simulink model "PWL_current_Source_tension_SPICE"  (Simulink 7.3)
settings: Solver=ode15s  StartTime=0.0  StopTime=10  RelTol=1e-3
StopFcn:
  | load signaux.mat
  | plotyy(x(1,:),x(2,:),x(1,:),x(3,:))
  | title('Dérivateur commandé par PWL Current et source I-->V')
  | xlabel('temps')
  | grid
  | gtext('Tension d''entrée')
  | gtext('Sortie du dérivateur')
libraries: fl_lib x10, nesl_utility x3, elec_lib x2

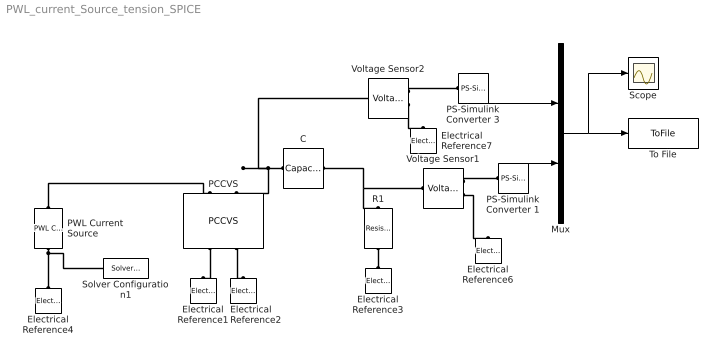
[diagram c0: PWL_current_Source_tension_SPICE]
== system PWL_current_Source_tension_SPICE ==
  C : fl_lib/Electrical/Electrical Elements/Capacitor  DialogController=NetworkEngine.DynNeDlgSource  SystemSampleTime=-1  c=1e-6 F  v0=0 V  r=0 Ohm  g=0 1/Ohm  i_Log=off  v_Log=off  vc_Log=off  LocalVarNames=|i|v|vc  LocalVarDescs=|i|v|Internal variable for voltage across capacitor term  LocalVarLogging=[0 0 0]
  Electrical Reference{1..4,6..7} (6 alike) : fl_lib/Electrical/Electrical Elements/Electrical Reference  DialogController=NetworkEngine.DynNeDlgSource  SystemSampleTime=-1  i_Log=off  LocalVarNames=|i  LocalVarDescs=|i  LocalVarLogging=[]
  Mux : Mux  Inputs=2
  PCCVS : elec_lib/Sources/SPICE-Compatible Sources/PCCVS  DialogController=NetworkEngine.DynNeDlgSource  SystemSampleTime=-1  PEES=[0 1 ]  LocalVarLogging=[]
  PS-Simulink Converter 1 : nesl_utility/PS-Simulink Converter  DialogController=NetworkEngine.DynNeUtilDlgSource  SystemSampleTime=-1  PhysicalDomain=network_engine_domain  LeftPortType=input  RightPortType=output  SubClassName=ps_output  Unit=1  AffineConversion=off
  PS-Simulink Converter 3 : nesl_utility/PS-Simulink Converter  DialogController=NetworkEngine.DynNeUtilDlgSource  SystemSampleTime=-1  PhysicalDomain=network_engine_domain  LeftPortType=input  RightPortType=output  SubClassName=ps_output  Unit=1  AffineConversion=off
  PWL Current Source : elec_lib/Sources/SPICE-Compatible Sources/PWL Current Source  DialogController=NetworkEngine.DynNeDlgSource  SystemSampleTime=-1  TIMElist=[0 1 2 3 4 5 6 7 8 9 10] s  CURRlist=[0 1 2 3 4 5 4 3 2 1 0] A  INTERP=1  EXTRAP=1  current_Log=off  voltage_Log=off  power_Log=off  LocalVarNames=|current|voltage|power  LocalVarDescs=|Current (A)|Voltage (V)|Power (W)  LocalVarLogging=[0 0 0]
  R1 : fl_lib/Electrical/Electrical Elements/Resistor  Tag=Factory Generic  DialogController=NetworkEngine.DynNeDlgSource  SystemSampleTime=-1  R=1 kOhm  i_Log=off  v_Log=off  LocalVarNames=|current|voltage|power  LocalVarDescs=|Resistor current (A)|Voltage across resistor (V)|Power (W)  LocalVarLogging=[0 0 0]
  Scope : Scope
  Solver Configuration1 : nesl_utility/Solver Configuration  DialogController=NetworkEngine.DynNeUtilDlgSource  SystemSampleTime=-1  PhysicalDomain=network_engine_domain  LeftPortType=input  RightPortType=generic  SubClassName=solver  Accelerate=off  Profile=off  ResidualTolerance=1e-9  MaxNonlinIter=12  MaxModeIter=2  DoFixedCost=off  DoDC=off  LinearAlgebra=Sparse
  To File : ToFile  Filename=signaux  MatrixName=x
  Voltage Sensor1 : fl_lib/Electrical/Electrical Sensors/Voltage Sensor  DialogController=NetworkEngine.DynNeDlgSource  SystemSampleTime=-1  i1_Log=off  v1_Log=off  LocalVarNames=|i1|v1  LocalVarDescs=|i1|v1  LocalVarLogging=[]
  Voltage Sensor2 : fl_lib/Electrical/Electrical Sensors/Voltage Sensor  DialogController=NetworkEngine.DynNeDlgSource  SystemSampleTime=-1  i1_Log=off  v1_Log=off  LocalVarNames=|i1|v1  LocalVarDescs=|i1|v1  LocalVarLogging=[]
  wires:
  PS-Simulink Converter 1/1 -> Mux/2
  Mux/1 -> To File/1, Scope/1
  PS-Simulink Converter 3/1 -> Mux/1
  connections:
  PWL Current Source/RConn1 -- Electrical Reference4/LConn1 -- Solver Configuration1/RConn1
  PCCVS/RConn1 -- Electrical Reference1/LConn1
  PCCVS/RConn2 -- Electrical Reference2/LConn1
  C/RConn1 -- Voltage Sensor2/LConn1 -- PCCVS/LConn2
  C/LConn1 -- Voltage Sensor1/LConn1 -- R1/LConn1
  R1/RConn1 -- Electrical Reference3/LConn1
  Voltage Sensor1/RConn1 -- PS-Simulink Converter 1/LConn1
  Voltage Sensor1/RConn2 -- Electrical Reference6/LConn1
  Voltage Sensor2/RConn1 -- PS-Simulink Converter 3/LConn1
  Voltage Sensor2/RConn2 -- Electrical Reference7/LConn1
  PWL Current Source/LConn1 -- PCCVS/LConn1
